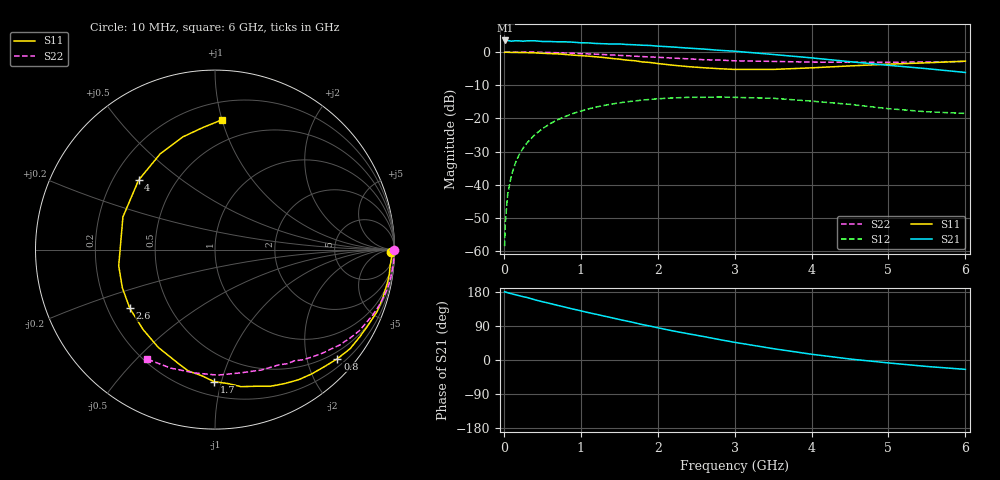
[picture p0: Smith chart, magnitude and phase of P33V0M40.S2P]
! SIEMENS Small Signal Semiconductors
! BFP181
! Si NPN RF Bipolar Junction Transistor in SOT143
! VCE = 3 V  IC = 0.4 mA
! Common Emitter S-Parameters:  March  1996
# GHz  S  MA  R  50
!  f  S11  S21  S12  S22
! GHz  MAG  ANG  MAG  ANG  MAG  ANG  MAG  ANG
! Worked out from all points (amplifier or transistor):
!   36 points, 10 MHz to 6 GHz, reference 50 ohm
!   highest |S21| = 3.4 dB at 20 MHz (marker M1)
!   |S21| within 3 dB of that: start of sweep to 2.827 GHz
!   unconditionally stable (mu >= 1): 3.861 GHz to end of sweep
!   at 250 MHz: K = 0.08, MSG = 16.1 dB, |S12| = -29.0 dB
!   at 1.4 GHz: K = 0.43, MSG = 9.0 dB, |S12| = -15.7 dB
!   at 6 GHz: K = 1.49, MAG = 2.0 dB, |S12| = -18.5 dB
!   S11 on the Smith chart (normalised r, x): 10 MHz: 75, -49; 800 MHz: 0.35, -2.58; 1.7 GHz: 0.30, -0.95; 2.6 GHz: 0.29, -0.29; 4 GHz: 0.31, +0.35; 6 GHz: 0.33, +1.00
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0.01  0.9814 -0.7  1.459 179.8  0.0012 83.8  0.9991 -0.2
0.02  0.9895 -1.1  1.484 179.7  0.0028 87.4  0.9988 -0.5
0.05  0.9856 -2.3  1.48 177.5  0.0072 89.3  0.9972 -1.3
0.1  0.98 -5.2  1.446 174.9  0.0142 85.5  0.9974 -2.6
0.15  0.9808 -7.9  1.469 172.2  0.0214 83.4  0.9976 -3.8
0.2  0.9786 -10.4  1.463 169.7  0.0286 82.7  0.9964 -5.1
0.3  0.9729 -15.9  1.465 165.1  0.0427 78.9  0.9935 -7.7
0.4  0.9669 -20.9  1.468 159.1  0.0564 75.2  0.9898 -10.2
0.6  0.9416 -31.2  1.431 149.2  0.083 67.4  0.9774 -15.2
0.8  0.9136 -41.7  1.416 139.3  0.1069 59.7  0.962 -20.0
1.1  0.8613 -57.4  1.364 125.0  0.1387 49.3  0.9318 -26.8
1.5  0.7771 -79.3  1.316 107.0  0.171 36.3  0.8858 -35.3
1.7  0.7355 -90.4  1.277 98.3  0.1827 30.4  0.8607 -39.3
1.9  0.6924 -102.3  1.248 89.6  0.1929 24.7  0.8383 -42.8
2.2  0.63 -120.1  1.183 76.7  0.203 16.8  0.8057 -48.0
2.6  0.5766 -145.4  1.101 61.8  0.2075 7.3  0.7612 -54.5
3  0.5441 -170.4  1.023 46.7  0.2071 -2.1  0.7342 -61.0
3.5  0.5443 160.5  0.914 30.0  0.2006 -11.5  0.7189 -69.0
4  0.5755 137.7  0.812 15.2  0.1818 -19.0  0.7011 -78.5
4.5  0.6149 119.7  0.712 2.6  0.1624 -24.7  0.6995 -88.8
5.5  0.6842 95.5  0.559 -17.1  0.1257 -22.7  0.7047 -110.5
6  0.7243 86.9  0.49 -24.7  0.1188 -17.9  0.7178 -121.7
